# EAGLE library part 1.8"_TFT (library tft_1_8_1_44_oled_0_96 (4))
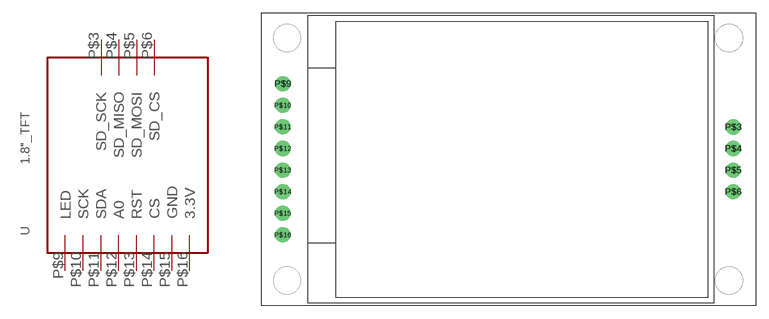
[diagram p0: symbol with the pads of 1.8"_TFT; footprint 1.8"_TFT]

Designator prefix -

## 1.8"_TFT  [1.8"_TFT]
P$3  SD_SCK
P$4  SD_MISO
P$5  SD_MOSI
P$6  SD_CS
P$9  LED
P$10  SCK
P$11  SDA
P$12  A0
P$13  RST
P$14  CS
P$15  GND
P$16  3.3V

## Footprint 1.8"_TFT (pad centres in mm)
1,8" TFT SPI 128*160 with SD
drill 1 pad 1.778: P$3 55.5,21.05; P$4 55.5,18.52; P$5 55.5,15.98; P$6 55.5,13.44; P$9 2.5,26.14; P$10 2.5,23.6; P$11 2.5,21.06; P$12 2.5,18.52; P$13 2.5,15.98; P$14 2.5,13.44; P$15 2.5,10.9; P$16 2.5,8.36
